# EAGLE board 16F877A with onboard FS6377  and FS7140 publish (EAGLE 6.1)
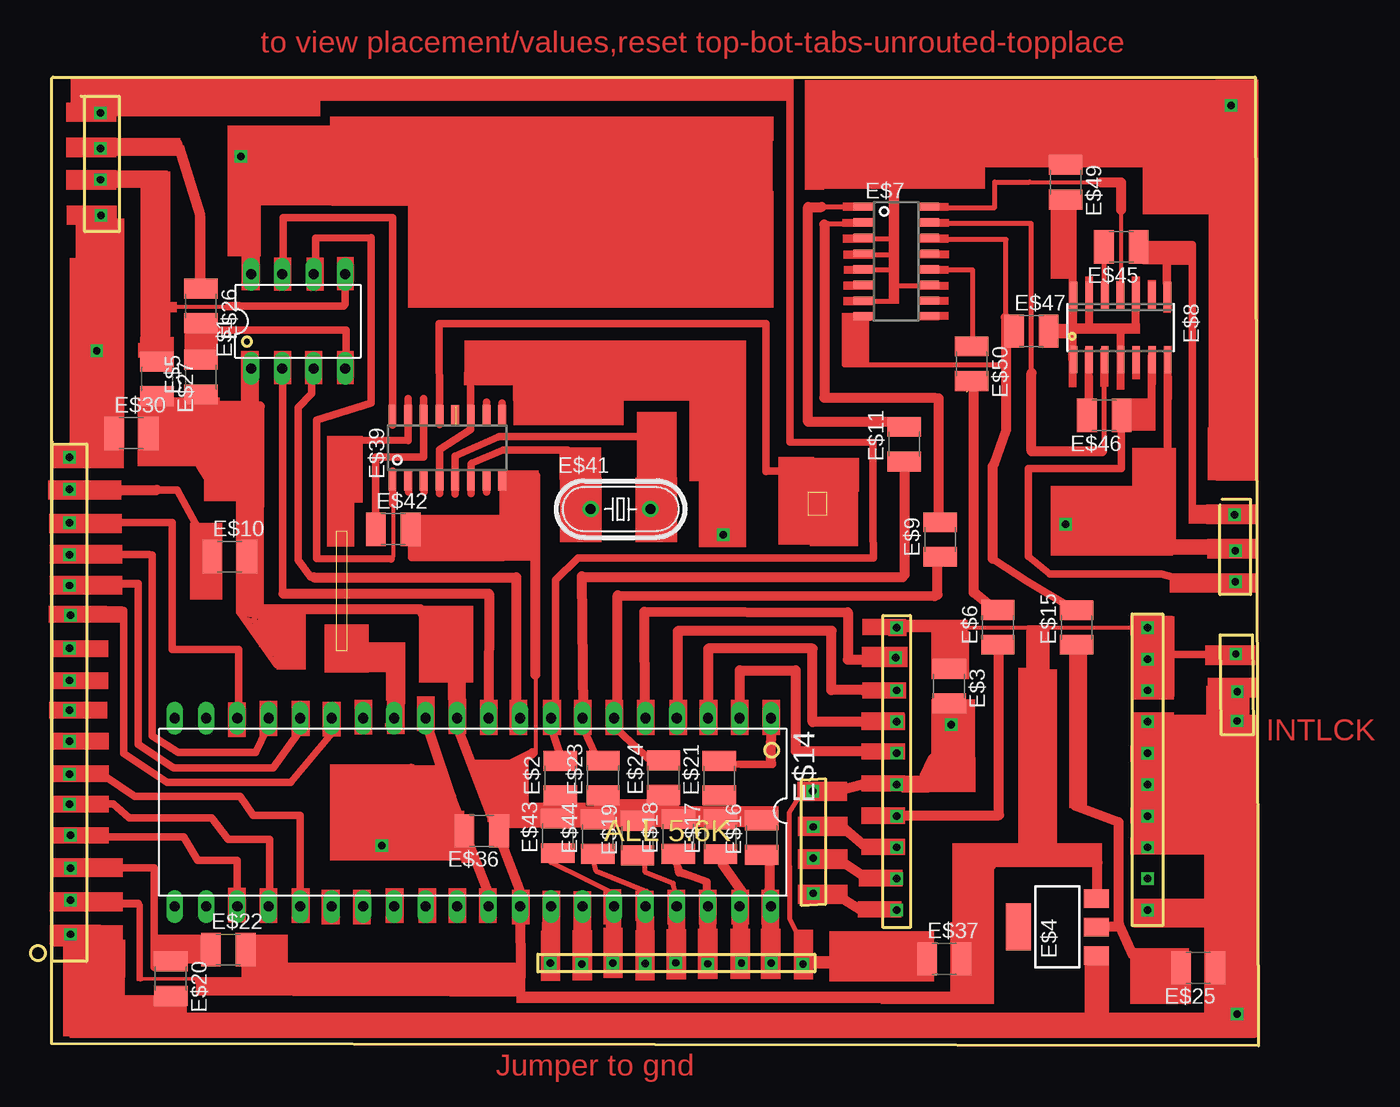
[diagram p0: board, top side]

Size 99.35 x 78.42 mm. Coordinates in mm from the lower left corner, seen from the top.
Outline: 4.05,76.88 4.36,76.88
Outline: 4.36,76.88 7.14,76.88 7.14,65.9 4.36,65.9 4.36,76.88
Outline: 96.4,44.26 98.71,44.26 98.71,36.52 96.24,36.52 96.24,43.79
Outline: 41.04,7.42 63.45,7.42 63.45,5.99 41.04,5.99 41.04,7.33
Outline: 62.46,21.54 64.29,21.64 64.29,11.45 62.38,11.36 62.38,21.46
Outline: 1.74,48.74 4.51,48.74 4.51,6.83 1.74,6.83 1.74,48.74
Outline: 1.74,48.74 1.74,48.89
Outline: 1.77,78.42 99.09,78.42 99.35,0 1.68,0.19 1.68,78.29
Outline: 96.25,33.28 98.87,33.28 98.96,25.19 96.34,25.19 96.25,33.28
Outline: 68.98,34.86 71.18,34.86 71.18,9.57 68.98,9.57 68.98,34.86
Outline: 89.13,34.98 91.59,34.98 91.59,9.73 89.13,9.73 89.13,34.98
Outline: circle at 84.27,57.43 radius 0.21
Outline: circle at 17.48,57.02 radius 0.36
Outline: circle at 59.97,23.95 radius 0.54
Outline: circle at 0.58,7.52 radius 0.58
Copper layers (1*16): Top 0.035mm / dielectric 1.5mm / Bottom 0.035mm
Design rules: minimum track width 10mil, minimum drill 24mil, track to track 8mil, track to pad 8mil, pad to pad 8mil, via to via 8mil, smd to smd 8mil, copper to edge 40mil, drill to drill 8mil, minimum pad ring 10mil, minimum via ring 8mil, stop-mask expansion 4mil, vias tented up to drill 0mil, thermal gap 10mil

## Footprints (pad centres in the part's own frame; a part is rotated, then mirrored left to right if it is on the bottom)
DIL08 = drill 0.813 long: 1 -3.81,-3.81; 2 -1.27,-3.81; 3 1.27,-3.81; 4 3.81,-3.81; 5 3.81,3.81; 6 1.27,3.81; 7 -1.27,3.81; 8 -3.81,3.81
C1210 = smd 1.6 x 2.7: 1 -1.4,0; 2 1.4,0
SOT223 = smd 1.5 x 2: 1 -2.3,-3.15; 2 0,-3.15; 3 2.3,-3.15 | smd 3.8 x 2: 4 0,3.15
SOIC16 = smd 0.635 x 1.524: 1 -4.445,-2.695; 2 -3.175,-2.695; 3 -1.905,-2.695; 4 -0.635,-2.695; 5 0.635,-2.695; 6 1.905,-2.695; 7 3.175,-2.695; 8 4.445,-2.695; 9 4.445,2.695; 10 3.175,2.695; 11 1.905,2.695; 12 0.635,2.695; 13 -0.635,2.695; 14 -1.905,2.695; 15 -3.175,2.695; 16 -4.445,2.695
SO14 = smd 0.6 x 2.2: 1 -3.81,-2.6; 2 -2.54,-2.6; 3 -1.27,-2.6; 4 0,-2.6; 5 1.27,-2.6; 6 2.54,-2.6; 7 3.81,-2.6; 8 3.81,2.6; 9 2.54,2.6; 10 1.27,2.6; 11 0,2.6; 12 -1.27,2.6; 13 -2.54,2.6; 14 -3.81,2.6
DIL40 = drill 0.813 long: 1 -24.13,-7.62; 2 -21.59,-7.62; 3 -19.05,-7.62; 4 -16.51,-7.62; 5 -13.97,-7.62; 6 -11.43,-7.62; 7 -8.89,-7.62; 8 -6.35,-7.62; 9 -3.81,-7.62; 10 -1.27,-7.62; 11 1.27,-7.62; 12 3.81,-7.62; 13 6.35,-7.62; 14 8.89,-7.62; 15 11.43,-7.62; 16 13.97,-7.62; 17 16.51,-7.62; 18 19.05,-7.62; 19 21.59,-7.62; 20 24.13,-7.62; 21 24.13,7.62; 22 21.59,7.62; 23 19.05,7.62; 24 16.51,7.62; 25 13.97,7.62; 26 11.43,7.62; 27 8.89,7.62; 28 6.35,7.62; 29 3.81,7.62; 30 1.27,7.62; 31 -1.27,7.62; 32 -3.81,7.62; 33 -6.35,7.62; 34 -8.89,7.62; 35 -11.43,7.62; 36 -13.97,7.62; 37 -16.51,7.62; 38 -19.05,7.62; 39 -21.59,7.62; 40 -24.13,7.62
HC49U-V = drill 0.813: 1 -2.413,0; 2 2.413,0

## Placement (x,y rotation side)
E$1  PIC 12F629  [DIL08]  21.62,58.64 0 top
E$2  5.6K  [C1210]  42.84,21.67 90 top
E$3  100NF  [C1210]  74.31,29.12 270 top
E$4  3.3V REG  [SOT223]  83.08,9.63 90 top
E$5  5.6K  [C1210]  13.76,54.14 90 top
E$6  ZERO  [C1210]  78.27,33.88 90 top
E$7  FS7140/5  [SOIC16]  70.04,63.51 270 top
E$8  74ALC74  [SO14]  88.19,58.16 180 top
E$9  100  [C1210]  73.6,40.99 90 top
E$10  100  [C1210]  16.1,39.6 0 top
E$11  100  [C1210]  70.67,48.71 90 top
E$14  [DIL40]  35.76,18.91 180 top
E$15  ZER0  [C1210]  84.63,33.87 90 top
E$16  5.6K  [C1210]  59.15,16.86 90 top
E$17  5.6K  [C1210]  55.82,16.93 90 top
E$18  5.6K  [C1210]  52.39,16.95 90 top
E$19  5.6K  [C1210]  49.1,16.82 90 top
E$20  470  [C1210]  11.32,5.45 270 top
E$21  5.6K  [C1210]  55.72,21.67 90 top
E$22  3.3K  [C1210]  15.98,7.8 0 top
E$23  5.6K  [C1210]  46.31,21.68 90 top
E$24  5.6K  [C1210]  51.2,21.72 90 top
E$25  47UFD  [C1210]  94.49,6.32 180 top
E$26  ZER0  [C1210]  13.76,59.9 270 top
E$27  5.6K  [C1210]  10.22,53.99 270 top
E$30  100NF  [C1210]  8.13,49.6 0 top
E$36  100NF  [C1210]  36.48,17.41 180 top
E$37  100NF  [C1210]  73.93,7.05 0 top
E$39  FS6377  [SOIC16]  33.7,48.42 0 top
E$41  16 MHZ  [HC49U-V]  47.72,43.45 0 top
E$42  ZERO  [C1210]  29.32,41.83 0 top
E$43  5.6K  [C1210]  42.65,17 90 top
E$44  5.6K  [C1210]  45.88,16.94 90 top
E$45  ZERO  [C1210]  88.25,64.67 180 top
E$46  ZERO  [C1210]  86.87,51.05 180 top
E$47  ZERO  [C1210]  80.97,57.86 0 top
E$49  100NF  [C1210]  83.74,69.91 270 top
E$50  ZERO  [C1210]  76.14,55.22 270 top

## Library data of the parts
E$1 E$14 = 74xx-eu
E$2 E$3 E$5 E$6 E$9-E$11 E$15-E$27 E$30 E$36 E$37 E$42-E$47 E$49 E$50 = resistor
E$4 = v-reg
E$7 E$39 = cypress
E$8 = analog-devices
E$41 = crystal

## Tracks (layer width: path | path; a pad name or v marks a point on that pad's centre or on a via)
S$1
  Top 0.61: 14.19,55.83 14.19,57.93 25.51,57.93 25.51,55.71
S$2
  Top 0.813: 31.52,35.35 18.49,35.35 18.52,51.78
S$3
  Top 0.61: 22.72,53.45 22.72,52.81 21.64,51.66 21.64,39.35 22.63,37.94
S$4
  Top 0.61: 42.15,25.65 42.96,23.24
S$5  (via drill 0.6)
  other vias: 5.33,56.27
S$6
  Top 0.61: 10.47,44.98 11.84,44.98 14.52,40.09
S$7
  Top 0.61: 10.48,55.71 10.48,59.79
S$8
  Top 0.61: 20.39,55.85 20.39,36.87
S$9
  Top 0.61: 17.65,54.84 17.65,51.63
S$10
  Top 0.813: 80.97,30.33 80.97,33.54
S$11
  Top 0.61: 7.51,35.26 7.51,23.68 11.04,21.33 21.02,21.33 24.37,25.33
S$12
  Top 0.813: 86.33,11.91 86.33,14.84 77.72,14.84 77.72,14.6
S$13
  Top 0.61: 6.28,70.05 10.48,70.05 10.48,59.66
S$14
  Top 0.813: 59.92,22.89 59.92,26.51
S$15  (via drill 0.6)
  other vias: 63.33,15.2
S$16  (via drill 0.6)
  other vias: 63.33,17.73
S$17  (via drill 0.6)
  other vias: 63.28,20.62
S$18  (via drill 0.6)
  other vias: 63.33,12.35
S$19
  Top 0.813: 65.58,20.74 67.28,21.16
S$20
  Top 0.813: 65.58,15 67.42,13.72
S$21
  Top 0.813: 65.65,17.76 67.56,16.13
S$22
  Top 0.813: 65.51,12.02 67.14,11.03
S$23
  Top 0.813: 4.59,48.15 4.59,55.65
S$24
  Top 0.61: 6.53,72.77 11.93,73.13 13.58,67.28 13.58,61.15
S$25
  Top 0.813: 20.44,36.62 37.07,36.61 37.05,27.4
S$26
  Top 0.813: 22.92,37.93 39.3,37.93 39.3,26.77
S$27
  Top 0.61: 42.46,27.71 42.46,37.71 44.3,39.49 61.33,39.48
S$28  (via drill 0.6)
  other vias: 97.12,76.11
S$29
  Top 0.61: 30.75,22.56 32.48,18.11 30.63,21.45 31.62,18.6 30.26,19.84
S$30  (via drill 0.6)
  other vias: 97.64,28.68
S$31
  Top 0.61: 20.41,62.65 20.41,67.03 29.26,67.03 29.26,54.21 29.26,50.25
S$32  (via drill 0.6)
  other vias: 97.64,2.6
S$33  (via drill 0.6)
  other vias: 97.52,31.73
S$34
  Top 0.813: 24.3,10.61 24.37,10.61
S$35  (via drill 0.6)
  other vias: 83.75,42.22
S$36
  Top 0.61: 93.99,42.98 93.99,64.84
S$37
  Top 1.016: 23.21,76.97 61.01,76.97
S$38
  Top 0.813: 88.06,9.87 88.04,18.1 84.5,19.44 84.56,31.7
S$39
  Top 0.406: 16.84,35.39 19.83,30.76 16.84,35.02 18.38,34.84 17.84,34.39 17.57,34.48 18.47,34.3 18.47,33.93 17.93,33.93 17.93,33.66 18.11,33.66 19.65,32.85 19.74,32.85 18.56,33.12
S$40  (via drill 0.6)
  other vias: 3.11,47.63
S$41  (via drill 0.6)
  other vias: 3.11,45.04
S$42  (via drill 0.6)
  other vias: 3.11,42.36
S$43
  Top 0.406: 39.71,5.48 39.74,10.53
S$44
  Top 0.813: 57.37,27.22 57.37,30.4 61.9,30.4 61.9,23.86 68.04,23.86
S$45
  Top 0.813: 68.04,26.22 63.27,26.21 63.27,32.16 54.81,32.16 54.81,27.22
S$46
  Top 0.813: 67.33,28.81 64.79,28.81 64.81,33.59 52.34,33.57 52.34,27.04
S$47
  Top 0.813: 49.72,26.94 49.66,35.15 66.11,35.09 66.11,31.28 68.36,31.28
S$48
  Top 0.813: 7.15,44.84 5.03,45.37
S$49
  Top 0.305: 8.87,5.44 39.68,5.51 39.68,5.43
S$50  (via drill 0.6)
  other vias: 3.11,39.77
S$51  (via drill 0.6)
  other vias: 3.11,37.27
S$52
  Top 0.61: 23.06,63.13 23.06,65.4 27.54,65.41 27.53,52.03 23.13,50.66 23.12,39.44 29.15,39.43
S$53
  Top 0.61: 33.06,44.71 33.06,48.29 35.6,49.89 35.6,54.88
S$54
  Top 0.61: 30.53,52.41 30.51,49.02 26.71,49.03
S$55
  Top 0.305: 40.84,29.85 40.84,23.62 40.55,23.6
S$56
  Top 0.61: 25.43,60.06 25.43,62.01
S$57  (via drill 0.6)
  other vias: 3.2,34.86
S$58
  Top 0.61: 83.32,42.05 83.32,40.04 95.59,40.04 95.59,40.25
S$59
  Top 0.61: 80.75,41.58 80.75,46.73 88.25,46.73 88.25,49.88
S$60  (1 unrouted)
S$61
  Top 0.61: 80.75,41.71 80.75,39.61 82.46,38.19 91.48,38.19 94.3,37.42 96.27,37.59
S$62  (via drill 0.6)
  other vias: 5.63,72.64
S$63
  Top 0.61: 77.97,39.32 80.66,37.59 83.95,35.62
S$64  (via drill 0.6)
  other vias: 3.11,32.17
S$65  (via drill 0.6)
  other vias: 3.11,29.58
S$66  (via drill 0.6)
  other vias: 5.63,70.12
S$68  (via drill 0.6)
  other vias: 3.11,27.17
S$69
  Top 0.813: 92.36,25.79 92.28,16.88
S$70  (via drill 0.6)
  other vias: 3.11,24.67
S$71  (via drill 0.6)
  other vias: 3.11,21.99
S$72  (via drill 0.6)
  other vias: 3.11,19.58
S$73  (via drill 0.6)
  other vias: 3.2,17.07
S$74  (via drill 0.6)
  other vias: 3.2,14.39
S$75  (via drill 0.6)
  other vias: 5.68,67.22
S$76  (via drill 0.6)
  other vias: 3.2,11.8
S$77
  Top 0.813: 77.85,39.43 77.84,46.92
S$78
  Top 0.305: 10.55,59.84 25.47,59.84
S$79  (via drill 0.6)
  other vias: 3.2,9.03
S$80  (via drill 0.6)
  other vias: 5.63,75.5
S$81
  Top 0.813: 44.58,38.04 44.69,26.99
S$82  (via drill 0.6)
  other vias: 97.63,26.31
S$83
  Top 0.813: 86.83,9.62 88.12,9.62 88.12,9.71 89.24,7.31
S$84
  Top 0.61: 97.7,31.61 95.81,31.69 93.95,31.67 91.73,31.67
S$85
  Top 0.61: 31.5,35.16 34.34,29.36 34.34,27.5
S$86
  Top 0.813: 73.46,52.41 73.46,42.54
S$87
  Top 0.813: 1.91,9.33 4.72,9.38
S$88
  Top 0.813: 73.39,36.54 73.39,39.22
S$89
  Top 0.61: 6.03,16.93 12.37,16.93 13.51,15.01 16.69,15.01 16.7,12.17
S$90
  Top 0.61: 6.95,42.35 11.42,42.35 11.42,32.08 16.83,32.08 16.8,27.21
S$91
  Top 0.813: 70.71,47.15 70.71,38.14
S$92
  Top 0.61: 31.79,52.41 31.79,47.68 27.89,47.66 27.89,41.79
S$93
  Top 0.61: 7.12,39.8 9.57,39.8
S$94
  Top 0.406: 6.82,37.32 8.63,37.32
S$95
  Top 0.406: 24.52,25.57 21.16,21.36 13.36,21.37
S$96
  Top 0.406: 9.86,39.66 9.86,25.06 11.72,23.74 18.23,23.74 18.83,25.16
S$97
  Top 0.61: 6.03,19.58 6.64,19.58 7.94,18.45 14.65,18.48 15.95,16.74 19.33,16.74 19.34,12.27
S$98  (via drill 0.6)
  other vias: 97.48,37.56
S$100  (via drill 0.6)
  other vias: 70.08,18.61
S$101
  Top 0.813: 17.8,62.07 17.8,64.4
S$102  (via drill 0.6)
  other vias: 70.08,21.15
S$103  (via drill 0.6)
  other vias: 70.08,23.69
S$104  (via drill 0.6)
  other vias: 70.08,10.99
S$105  (via drill 0.6)
  other vias: 70.08,26.23
S$106  (via drill 0.6)
  other vias: 70.08,13.53
S$107  (via drill 0.6)
  other vias: 70.08,16.07
S$108  (via drill 0.6)
  other vias: 70.08,28.77
S$109  (via drill 0.6)
  other vias: 90.4,28.77
S$110  (via drill 0.6)
  other vias: 90.4,23.69
S$111  (via drill 0.6)
  other vias: 90.4,26.23
S$112  (via drill 0.6)
  other vias: 90.4,21.15
S$113  (via drill 0.6)
  other vias: 90.4,18.61
S$114  (via drill 0.6)
  other vias: 90.4,16.07
S$116  (via drill 0.6)
  other vias: 90.4,13.53
S$117  (via drill 0.6)
  other vias: 70.08,13.53
S$118  (via drill 0.6)
  other vias: 70.08,26.23
S$119  (via drill 0.6)
  other vias: 70.08,18.61
S$120  (via drill 0.6)
  other vias: 90.4,31.31
S$121  (via drill 0.6)
  other vias: 70.08,33.85
S$122  (via drill 0.6)
  other vias: 90.4,23.69
S$123  (via drill 0.6)
  other vias: 90.4,10.99
S$124  (via drill 0.6)
  other vias: 90.4,21.15
S$125  (via drill 0.6)
  other vias: 70.08,21.15
S$126  (via drill 0.6)
  other vias: 90.4,13.53
S$127  (via drill 0.6)
  other vias: 70.08,23.69
S$128  (via drill 0.6)
  other vias: 70.08,28.77
S$129  (via drill 0.6)
  other vias: 90.4,26.23 70,31.42
S$130  (via drill 0.6)
  other vias: 90.4,33.85
S$131  (via drill 0.6)
  other vias: 90.4,28.77
S$132  (via drill 0.6)
  other vias: 90.4,18.61
S$133  (via drill 0.6)
  other vias: 90.4,16.07
S$134
  Top 0.813: 69.99,33.79 69.99,33.89
S$135
  Top 0.406: 5.23,8.34 5.11,8.34
S$136
  Top 0.813: 90.42,26.2 90.42,26.07
S$137
  Top 0.813: 86.48,2.39 86.48,6.98
S$138
  Top 0.305: 75.7,33.86 90.14,33.86 90.14,34.36
S$139
  Top 0.61: 16.79,59.87 25.3,59.87
S$140  (via drill 0.6)
  other vias: 16.99,71.99
S$141
  Top 0.813: 44.71,37.94 70.55,37.94
S$142
  Top 0.813: 90.31,33.84 90.31,33.66
S$143
  Top 0.61: 38.26,45.22 40.81,45.22 40.81,39
S$144
  Top 0.61: 35.61,47.08 35.61,44.72
S$145
  Top 0.813: 47.05,27.11 47.49,27.11 47.49,36.47 73.14,36.41
S$146
  Top 0.813: 11.96,72.77 13.69,67.21 13.69,61.89
S$147
  Top 0.406: 68.35,33.83 68.35,33.99
S$148
  Top 0.813: 59.99,26.89 59.96,26.89
S$149
  Top 0.813: 70.34,16.1 70.34,16.21
S$150
  Top 0.813: 77.51,35.74 76.32,36.7 76.32,53.22
S$151
  Top 0.813: 54.7,26.26 54.91,26.26
S$152
  Top 0.813: 70.12,18.65 78.36,18.66 78.36,32.21
S$153  (via drill 0.6)
  other vias: 28.39,16.21
S$155
  Top 0.813: 37.89,22.33 40.58,23.69
S$156
  Top 0.813: 29.81,25.97 29.07,25.97
S$158  (via drill 0.6)
  other vias: 97.48,40.08
S$159
  Top 0.813: 40.83,30.05 40.84,46.15
S$160
  Top 0.813: 32.03,26.07 34.33,19.2
S$161
  Top 0.813: 37.21,11.96 34.02,20.16
S$162
  Top 0.813: 34.58,25.6 39.85,11.87
S$163
  Top 0.813: 59.77,14.96 59.77,12.64
S$164
  Top 0.406: 6.78,11.39 8.87,11.39 8.87,5.41
S$165
  Top 0.406: 7.24,14.35 9.96,14.35 9.96,8.4 | 10.3,8.31 9.96,8.4 | 9.96,8.4 14.72,8.4
S$166
  Top 0.406: 17.96,7.55 20.51,7.55 20.51,5.33
S$167
  Top 0.813: 69.35,23.84 69.35,23.63
S$168
  Top 0.61: 35.7,47.2 38.2,48.23 43.3,48.25
S$169
  Top 0.61: 34.35,44.69 34.35,47.76 37.8,49.28
S$170
  Top 0.813: 39.59,11.13 39.61,5.5
S$171
  Top 0.61: 33.07,50.28 33.06,58.47 59.48,58.45 59.48,46.49
S$172
  Top 0.61: 31.81,39.55 38.22,39.55 38.22,45.66
S$173
  Top 0.61: 43.42,48.23 43.44,45.88
S$174  (1 unrouted)
  Top 0.61: 36.88,50.69 36.88,52.09 | 38.14,50.64 38.14,52.05 | 36.88,44.83 36.88,46.24 | 31.83,44.85 31.83,46.26 | 30.56,44.85 30.56,46.33 | 29.28,43.87 29.28,46.53
S$175
  Top 0.61: 37.94,49.31 50.75,49.31
S$176
  Top 0.61: 7.28,37.43 8.69,37.43 8.69,24.39 11.57,22.51 19.61,22.51 21.61,25.27
S$178
  Top 0.61: 9.8,39.72 9.8,25.09 11.92,23.74 18.2,23.74 19.08,25.62
S$179
  Top 0.61: 31.69,39.55 30.82,39.55 30.87,41.5
S$180
  Top 0.305: 29.32,45.72 29.33,39.64
S$181  (via drill 0.6)
  other vias: 56.02,41.37
S$185
  Top 0.61: 61.42,77.22 61.42,48.89 68.17,48.85 68.17,42.03 68.19,39.48 61.16,39.49
S$186
  Top 0.61: 59.54,46.52 63.83,46.52
S$187
  Top 0.406: 49.84,12.52 45.73,14.18 45.43,15.49
S$188  (via drill 0.6)
  other vias: 97.43,42.98
S$189
  Top 0.406: 47.16,12.34 44.9,13.47 42.1,14.84 41.86,15.37
S$190
  Top 0.406: 52.17,12.34 51.99,13.17 49.72,14.06 49.72,14.72
S$191
  Top 0.406: 84.37,53.92 84.37,62.35
S$192
  Top 0.406: 84.49,57.98 88.2,57.98 88.2,55.93
S$193
  Top 0.406: 85.58,59.79 85.58,58.14
S$194
  Top 0.406: 89.42,59.47 89.42,58 87.95,58
S$195
  Top 0.406: 91.86,61.32 91.94,61.32
S$196
  Top 0.406: 88.18,60.61 88.28,60.61
S$197
  Top 0.406: 86.89,48.14 86.87,54.35
S$198
  Top 0.406: 86.87,61.43 86.9,64.18
S$199
  Top 0.406: 92,61.28 92,64.66 92.05,64.9 89.8,64.9 89.72,64.86
S$200
  Top 0.406: 85.66,50.5 85.66,54.18 | 85.36,50.13 85.36,50.31
S$201
  Top 0.406: 90.82,54.31 90.82,51.42 90.6,51.44 90.6,51.29 88.7,51.29
S$202
  Top 0.813: 80.98,54.47 80.98,48.14 86.68,48.14
S$203
  Top 0.406: 92.02,64.93 93.39,64.93
S$205
  Top 0.813: 89.92,64.94 89.92,64.85
S$206
  Top 0.813: 95.47,72.38 95.43,67.69
S$207
  Top 0.406: 19.71,22.63 21.78,25.47
S$208
  Top 0.406: 84.4,61.27 84.4,68.01
S$209
  Top 0.61: 52.27,14.78 52.52,14.11 54.72,13.28 54.72,12.56
S$210
  Top 0.305: 80.58,69.9 88.22,69.9 88.22,61.33
S$211
  Top 0.813: 86.62,69.9 88.22,69.9 88.22,67.68
S$212
  Top 0.813: 5.96,14.15 5.96,14.11
S$213
  Top 0.813: 89.1,51.04 89.1,51.31 90.42,51.31
S$215
  Top 0.61: 90.12,64.84 93.86,64.84
S$216
  Top 0.813: 55.99,14.68 57.66,12.32
S$217
  Top 0.406: 54.6,11.8 54.6,13.27 52.38,13.91 52.17,14.96
S$218
  Top 0.406: 62.1,20.03 61.36,18.87 61.4,10.33 62.1,8.97
S$219  (via drill 0.6)
  other vias: 57.51,6.7
S$220  (via drill 0.6)
  other vias: 54.78,6.65
S$221  (via drill 0.6)
  other vias: 52.19,6.73
S$222  (via drill 0.6)
  other vias: 59.92,6.7
S$223  (via drill 0.6)
  other vias: 47.11,6.71
S$224  (via drill 0.6)
  other vias: 44.59,6.63
S$225  (via drill 0.6)
  other vias: 42.03,6.71
S$226  (via drill 0.6)
  other vias: 49.71,6.66
S$227  (via drill 0.6)
  other vias: 62.49,6.63
S$228
  Top 1.016: 63.28,6.75 72.67,6.75
S$229
  Top 0.61: 14.45,45.74 13.67,46.94
S$230
  Top 0.406: 88.29,47.86 88.29,49.81
S$231
  Top 0.813: 6.79,45.01 10.21,45.01
S$232
  Top 0.813: 78.91,58.97 78.91,49.85 77.94,47.1
S$233
  Top 0.406: 64.5,66.57 66.73,66.57
S$234
  Top 0.406: 63.58,67.94 67.15,67.94
S$235
  Top 0.305: 68.81,4.1 75.44,4.1
S$240
  Top 1.27: 73.15,23.1 72.53,21.74
S$242
  Top 0.61: 44.78,25.57 46.11,22.65
S$243
  Top 1.27: 6.41,62.58 6.62,61.86
S$244
  Top 0.61: 47.4,25.65 50.3,22.97
S$245
  Top 0.61: 60.01,22.78 57.47,22.78 54.86,22.83
S$255  (1 unrouted)
S$258
  Top 0.813: 64,67.9 62.91,67.9 62.91,50.5 71.11,50.5
S$269
  Top 0.406: 73.37,62.83 76.22,62.83 76.22,57.12
S$270
  Top 0.406: 69.82,61.88 69.82,62.84 67.79,62.84
S$271  (via drill 0.6)
  other vias: 74.48,25.99
S$272
  Top 0.61: 6.03,21.81 8.39,20.19 16.96,20.19 17.99,18.67 21.78,18.67 21.79,12.39
S$273
  Top 0.406: 13.35,21.36 11.01,21.41 7.59,23.75 7.59,34.67
S$274
  Top 0.406: 6.57,34.94 7.54,34.67
S$275
  Top 0.61: 6.98,14.4 9.92,14.4
S$276
  Top 0.61: 6.51,11.52 8.69,11.52
S$277
  Top 0.61: 9.98,14.4 9.98,6.35
S$278
  Top 0.406: 67.67,64.03 69.7,64.03
S$279
  Top 0.406: 70.09,61.54 72.01,61.54
S$280
  Top 0.406: 72.79,67.86 78.01,67.86 78.01,69.92 80.83,69.92
S$281
  Top 0.406: 73.28,66.57 80.96,66.57 80.96,54.47
S$282
  Top 0.406: 67.66,59.03 65.82,59.03 65.82,55.13 78.59,55.13 78.59,55.05
S$283
  Top 0.406: 73.12,65.29 78.92,65.29 78.92,57.87
S$284
  Top 0.406: 66.57,65.33 69.97,65.33
S$291
  Top 0.406: 66.57,60.27 69.8,60.27 69.8,61.6
S$292
  Top 0.813: 64.22,66.49 64.22,52.47 73.16,52.47
(copper drawn outside any net)
  shapes: Top area x328

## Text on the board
Top: to view placement/values,reset top-bot-tabs-unrouted-topplace | FS7140 OR FS7145 | pin 1 | INTLCK | Jumper to gnd
Dimension: ALL 5.6K
tValues: PB | GND | GND | ROT A | PIN 1 | ROT B | GND | GND | PIN 1 | PIN 1 | PIN 1 | GND | I | GND | JUMPER | GND | PIN 1 | Q | JUMPER | +5 VOLT | GND | PIN 1 | GND | 16F877A | GND | GND | SQR | 16 X 2 LCD DISPLAY | SINE NO FILTER | SINE W-LPF | PIN 1 | GND | GND | DN5KHZ | UP5KHZ | BANDSW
